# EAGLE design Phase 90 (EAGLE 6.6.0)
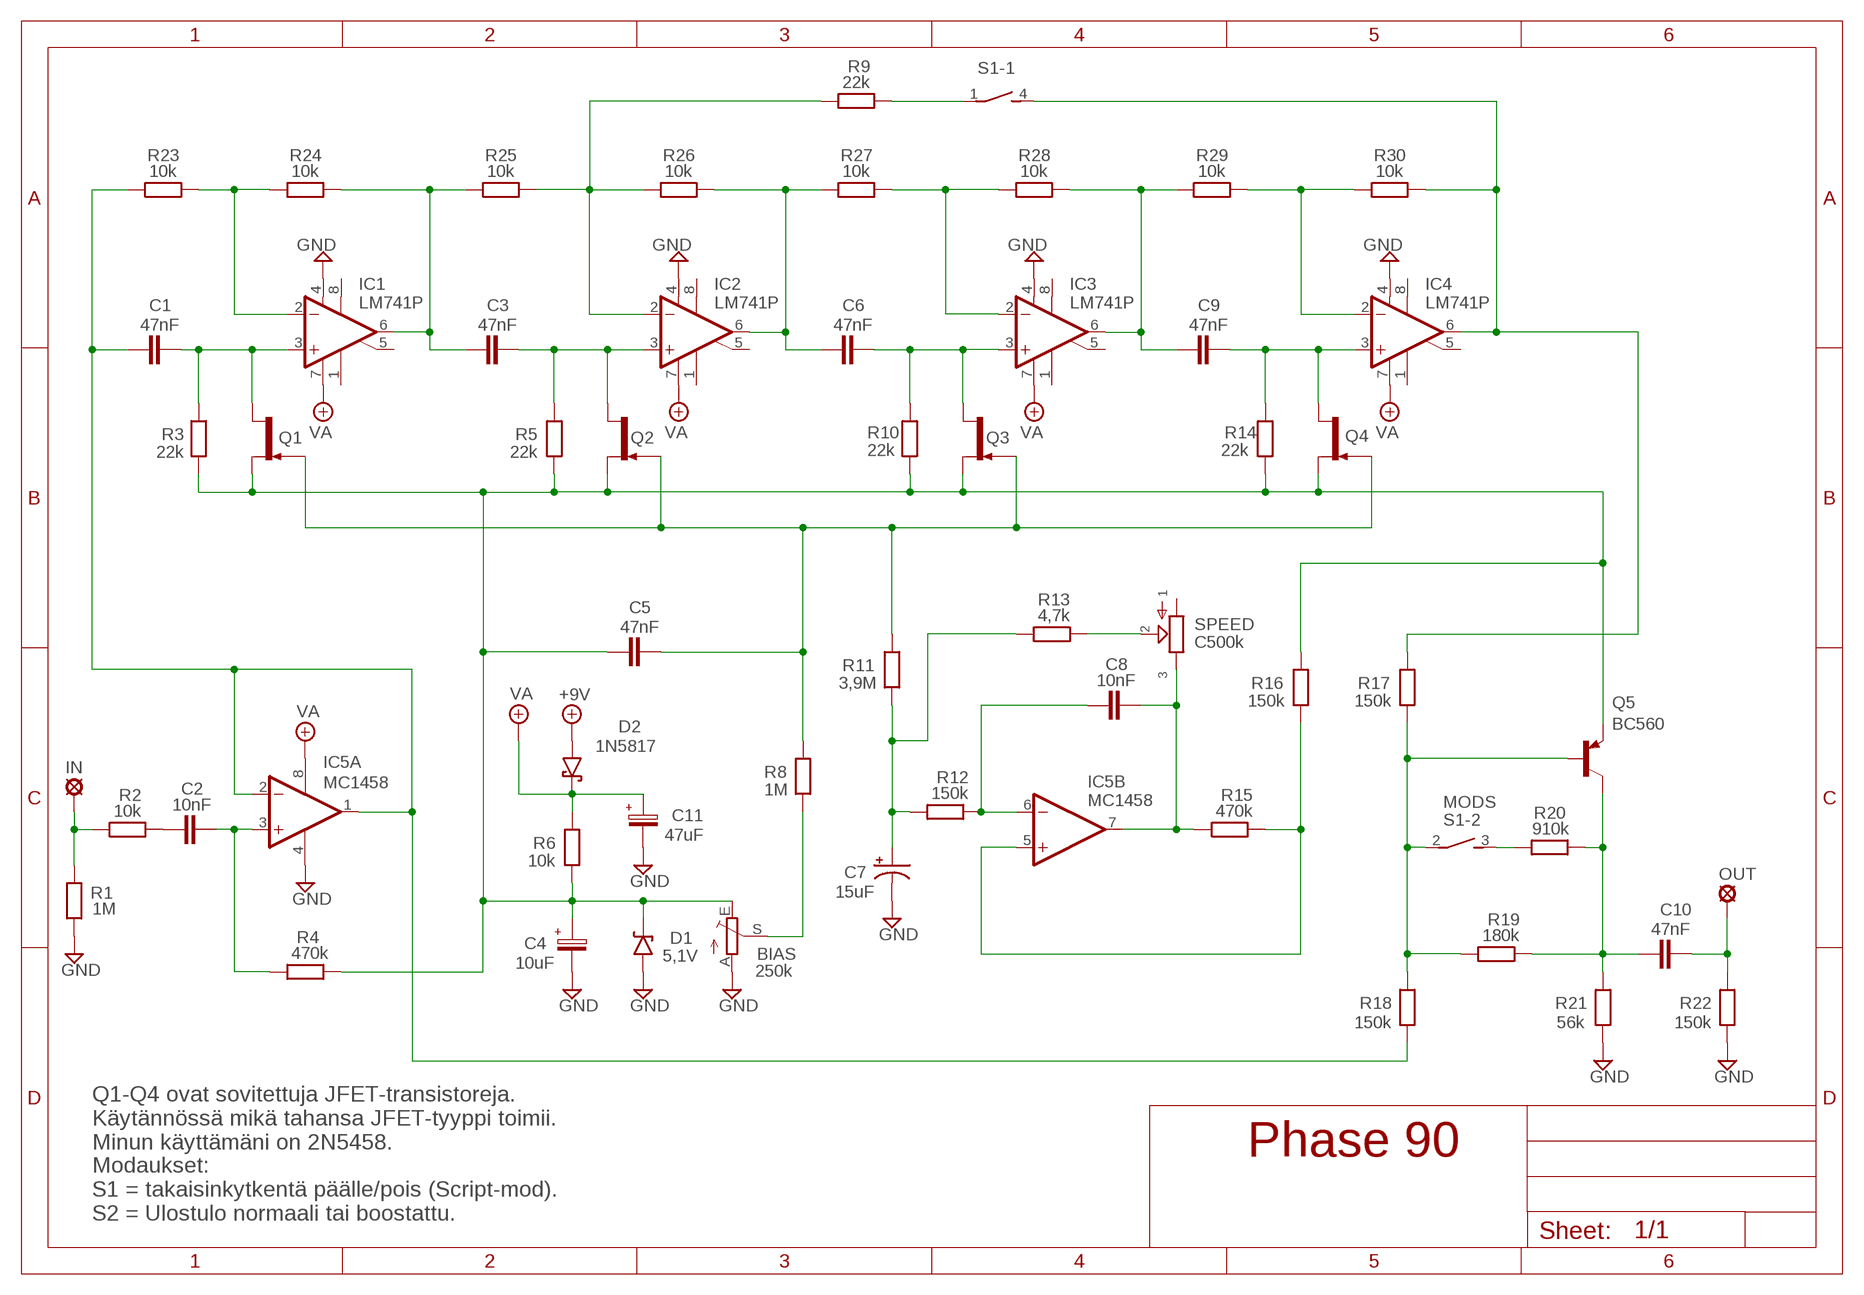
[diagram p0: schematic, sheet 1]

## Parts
+9V  +9V  +9V(T)1  [ROUND]
BIAS  250k  TRIM_EU-PT10  [PT-10]
C1  47nF  22NF-82NF"  [4,5MM]
C2  10nF  1NF-15NF  [3,5MM]
C3  47nF  22NF-82NF"  [4,5MM]
C4  10uF  063-EU  [063_025]
C5  47nF  22NF-82NF"  [4,5MM]
C6  47nF  22NF-82NF"  [4,5MM]
C7  15uF  044A2  [044A_2]
C8  10nF  1NF-15NF  [3,5MM]
C9  47nF  22NF-82NF"  [4,5MM]
C10  47nF  22NF-82NF"  [4,5MM]
C11  47uF  063-EU  [063_025]
D1  5,1V  1N9ZENER  [DO35-3]
D2  1N5817  [DO41-3]
GND  GND  GND(T)1  [ROUND]
GND5  GND  GND(T)1  [ROUND]
IC1  LM741P  [DIL08]
IC2  LM741P  [DIL08]
IC3  LM741P  [DIL08]
IC4  LM741P  [DIL08]
IC5  MC1458  TL072P  [DIL08]
IN  MCS10B  [MCS10B]
OUT  MCS10B  [MCS10B]
Q1  2N5457  [TO92-]
Q2  2N5457  [TO92-]
Q3  2N5457  [TO92-]
Q4  2N5457  [TO92-]
Q5  BC560  [TO92-EBC]
R1  1M  6MM-EU3  [R0207/3]
R2  10k  6MM-EU3  [R0207/3]
R3  22k  6MM-EU3  [R0207/3]
R4  470k  6MM-EU3  [R0207/3]
R5  22k  6MM-EU3  [R0207/3]
R6  10k  6MM-EU3  [R0207/3]
R8  1M  6MM-EU3  [R0207/3]
R9  22k  6MM-EU3  [R0207/3]
R10  22k  6MM-EU3  [R0207/3]
R11  3,9M  6MM-EU3  [R0207/3]
R12  150k  6MM-EU3  [R0207/3]
R13  4,7k  6MM-EU3  [R0207/3]
R14  22k  6MM-EU3  [R0207/3]
R15  470k  6MM-EU3  [R0207/3]
R16  150k  6MM-EU3  [R0207/3]
R17  150k  6MM-EU3  [R0207/3]
R18  150k  6MM-EU3  [R0207/3]
R19  180k  6MM-EU3  [R0207/3]
R20  910k  6MM-EU3  [R0207/3]
R21  56k  6MM-EU3  [R0207/3]
R22  150k  6MM-EU3  [R0207/3]
R23  10k  6MM-EU3  [R0207/3]
R24  10k  6MM-EU3  [R0207/3]
R25  10k  6MM-EU3  [R0207/3]
R26  10k  6MM-EU3  [R0207/3]
R27  10k  6MM-EU3  [R0207/3]
R28  10k  6MM-EU3  [R0207/3]
R29  10k  6MM-EU3  [R0207/3]
R30  10k  6MM-EU3  [R0207/3]
S1  MODS  DS02E  [DS-02]
SPEED  C500k  POT-EU16MM  [16MM]

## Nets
+9V: +9V.1(+9V) D2.A
GND: BIAS.A C4.- C7.2(-) C11.- D1.A GND5.1(GND) GND.1(GND) IC1.4(V-) IC2.4(V-) IC3.4(V-) IC4.4(V-) IC5.4(P:V-) R1.1 R21.1 R22.1
N$1: IC1.2(-IN) R23.2 R24.1
N$2: C1.2 IC1.3(+IN) Q1.3(D) R3.2
N$3: IC2.2(-IN) R9.1 R25.2 R26.1
N$4: C5.2 Q1.1(G) Q2.1(G) Q3.1(G) Q4.1(G) R8.2 R11.2
N$5: R20.1 S1.3
N$6: IC3.2(-IN) R27.2 R28.1
N$7: C3.1 IC1.6(OUT) R24.2 R25.1
N$8: C3.2 IC2.3(+IN) Q2.3(D) R5.2
N$9: R9.2 S1.1
N$10: C6.1 IC2.6(OUT) R26.2 R27.1
N$11: IC4.2(-IN) R29.2 R30.1
N$12: BIAS.S R8.1
N$13: C6.2 IC3.3(+IN) Q3.3(D) R10.2
N$14: C10.1 Q5.C R19.2 R20.2 R21.2
N$15: C9.2 IC4.3(+IN) Q4.3(D) R14.2
N$16: C9.1 IC3.6(OUT) R28.2 R29.1
N$17: IN.MP R1.2 R2.1
N$18: IC4.6(OUT) R17.2 R30.2 S1.4
N$19: C2.1 R2.2
N$20: C2.2 IC5.3(A:+IN) R4.1
N$21: C1.1 IC5.1(A:OUT) IC5.2(A:-IN) R18.1 R23.1
N$22: C10.2 OUT.MP R22.2
N$23: C8.2 IC5.7(B:OUT) R15.1 SPEED.3
N$24: IC5.5(B:+IN) R15.2 R16.1
N$25: C8.1 IC5.6(B:-IN) R12.2
N$26: C7.1(+) R11.1 R12.1 R13.1
N$27: R13.2 SPEED.2
N$28: Q5.B R17.1 R18.2 R19.1 S1.2
N$29: BIAS.E C4.+ C5.1 D1.C Q1.2(S) Q2.2(S) Q3.2(S) Q4.2(S) Q5.E R3.1 R4.2 R5.1 R6.1 R10.1 R14.1 R16.2
VA: C11.+ D2.C IC1.7(V+) IC2.7(V+) IC3.7(V+) IC4.7(V+) IC5.8(P:V+) R6.2
Unconnected: IC1.1(ON1) IC1.5(ON2) IC1.8(OPT) IC2.1(ON1) IC2.5(ON2) IC2.8(OPT) IC3.1(ON1) IC3.5(ON2) IC3.8(OPT) IC4.1(ON1) IC4.5(ON2) IC4.8(OPT) SPEED.1

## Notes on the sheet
- Q1-Q4 ovat sovitettuja JFET-transistoreja. 
  Käytännössä mikä tahansa JFET-tyyppi toimii.
  Minun käyttämäni on 2N5458.
- Modaukset:
  S1 = takaisinkytkentä päälle/pois (Script-mod).
  S2 = Ulostulo normaali tai boostattu.

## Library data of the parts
+9V = gm-supply:+9V(T): +9V Voltage Supply
BIAS = pot:TRIM_EU-: POTENTIOMETER
C1 C3 C5 C6 C9 C10 = Mylar Kondensaattorit:22NF-82NF: 22nF-82nF
C2 C8 = Mylar Kondensaattorit:1NF-15NF: 1nF-15nF
C4 C11 = Elektrolyytit:063-EU
C7 = Tantaalit:044A: .1 - 1.5µF
D1 = Diodit:1N9*ZENER: 1N9???B Zener Diode
D2 = Diodit:1N5817
GND GND5 = gm-supply:GND(T): Ground
IC1-IC4 = Operaatiovahvistimet:*741: OP AMP
IC5 = Operaatiovahvistimet:TL072: OP AMP
IN OUT = Padit:MCS10B: SOLDER PAD
Q1-Q4 = Transistorit:2N5457: N-CHANNEL JFET
Q5 = transistor-pnp:BC560*: PNP Transistror
R1-R6 R8-R30 = Vastukset:6MM-EU: 6mm Resistors (European schematic symbol)
S1 = switch-dil:DS02E: DIL/CODE SWITCH; OC_FARNELL: 9472126; OC_NEWARK: unknown
SPEED = gm-pots:POT-EU

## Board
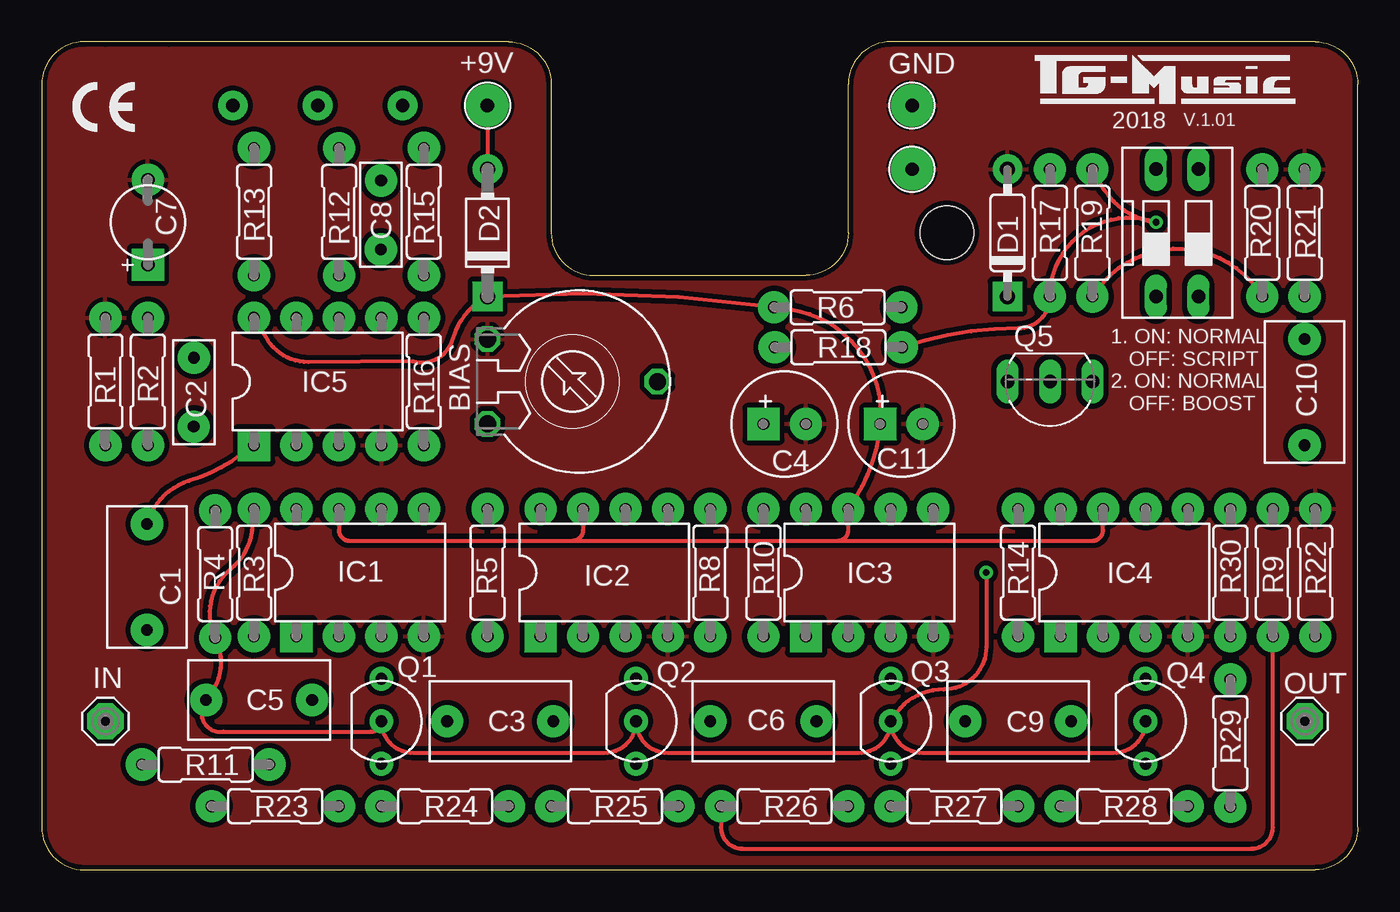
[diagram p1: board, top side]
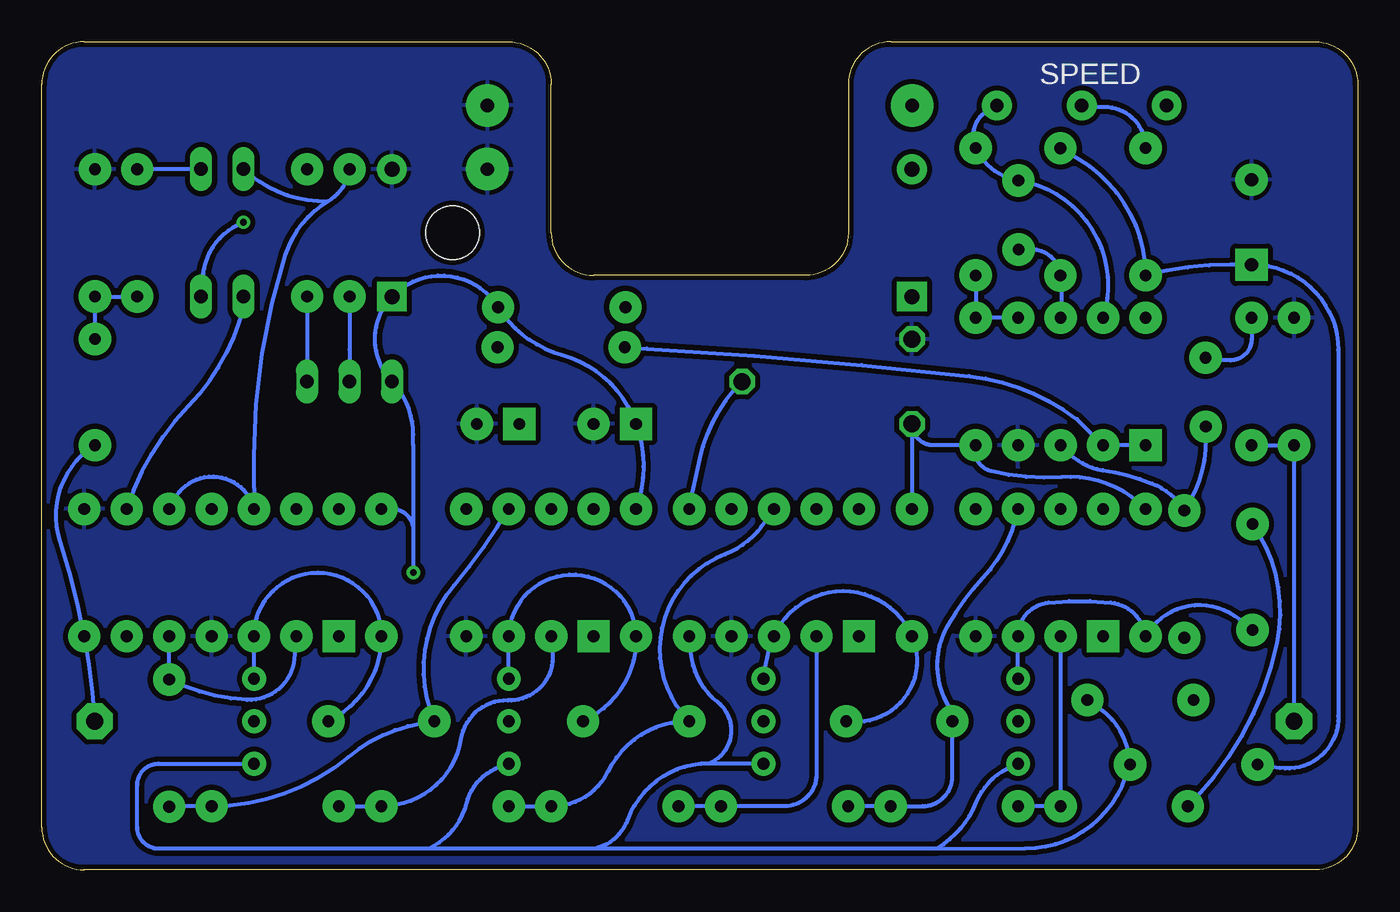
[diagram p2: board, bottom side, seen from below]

Size 78.74 x 49.53 mm. Coordinates in mm from the lower left corner, seen from the top.
Outline: 7.62,49.53 3.81,49.53
Outline: 78.74,2.54 78.74,46.99 arc90 76.2,49.53 50.8,49.53 arc90 48.26,46.99 48.26,38.1 arc-90 45.72,35.56 33.02,35.56 arc-90 30.48,38.1 30.48,46.99 arc90 27.94,49.53 2.54,49.53 arc90 0,46.99 0,2.54 arc90 2.54,0 76.2,0 arc90 78.74,2.54
Copper layers (1*16): Top 0.035mm / dielectric 1.5mm / Bottom 0.035mm
Design rules "ITEADstudio": minimum track width 10mil, minimum drill 12mil, track to track 12mil, track to pad 12mil, pad to pad 12mil, via to via 12mil, smd to smd 0mil, copper to edge 12mil, drill to drill 12mil, minimum pad ring 10mil, minimum via ring 6mil, stop-mask expansion 4mil, vias tented up to drill 100mil, thermal gap 10mil
Holes 3.2 mm at 54.16,38.11

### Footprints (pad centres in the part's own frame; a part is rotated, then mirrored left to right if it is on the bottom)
ROUND = drill 0.8 pad 2.54: 1 0,0
PT-10 = drill 1.016 octagon: A -2.54,-5.08; E 2.54,-5.08; S 0,5.08
4,5MM = drill 0.7 pad 1.93: 1 -3.175,0; 2 3.175,0
3,5MM = drill 0.7 pad 1.93: 1 -1.905,0; 2 2.221,-0.016
063_025 = drill 0.7 pad 1.93 square: + -1.27,0 | drill 0.7 pad 1.93: - 1.27,0
044A_2 = drill 0.8 pad 1.93 square: 1 -2.54,0 | drill 0.8 pad 1.93: 2 2.54,0
DO35-3 = drill 0.9 pad 1.778: A 3.81,0 | drill 0.9 pad 1.778 square: C -3.81,0
DO41-3 = drill 0.9 pad 1.778: A 3.81,0 | drill 0.9 pad 1.778 square: C -3.81,0
DIL08 = drill 0.7 pad 1.93 square: 1 -3.81,-3.81 | drill 0.7 pad 1.93: 2 -1.27,-3.81; 3 1.27,-3.81; 4 3.81,-3.81; 5 3.81,3.81; 6 1.27,3.81; 7 -1.27,3.81; 8 -3.81,3.81
MCS10B = drill 1.016 pad 2.159 octagon: MP 0,0
TO92- = drill 0.7 pad 1.422: 1 2.54,0; 2 0,0; 3 -2.54,0
TO92-EBC = drill 0.813 long: B 0,-1.27; C -2.54,-1.27; E 2.54,-1.27
R0207/3 = drill 0.7 pad 1.93: 1 -3.81,0; 2 3.81,0
DS-02 = drill 0.813 long: 1 -1.27,-3.81; 2 1.27,-3.81; 3 1.27,3.81; 4 -1.27,3.81
16MM = drill 0.8 pad 1.778: 1 5.08,0; 2 0,0; 3 -5.08,0

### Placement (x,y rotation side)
+9V  26.67,45.72 0 top
BIAS  31.75,29.21 270 top
C1  6.3,17.51 270 top
C2  9.11,28.73 270 top
C3  27.43,8.89 0 top
C4  44.45,26.67 0 top
C5  13.01,10.16 0 top
C6  43.18,8.89 0 top
C7  6.35,38.73 90 top
C8  20.29,39.02 90 top
C9  58.42,8.89 0 top
C10  75.56,28.57 270 top
C11  51.44,26.67 0 top
D1  57.78,38.1 90 top
D2  26.67,38.1 90 top
GND  52.07,45.72 0 top
GND5  52.07,41.91 0 top
IC1  19.05,17.78 0 top
IC2  33.66,17.78 0 top
IC3  49.53,17.78 0 top
IC4  64.77,17.78 0 top
IC5  16.51,29.21 0 top
IN  3.81,8.89 0 top
OUT  75.56,8.89 0 top
Q1  20.32,8.89 270 top
Q2  35.56,8.89 270 top
Q3  50.8,8.89 270 top
Q4  66.04,8.89 270 top
Q5  60.33,27.94 180 top
R1  3.81,29.21 270 top
R2  6.35,29.21 90 top
R3  12.7,17.78 270 top
R4  10.38,17.69 270 top
R5  26.67,17.78 270 top
R6  47.62,33.66 180 top
R8  40.01,17.78 270 top
R9  73.66,17.78 90 top
R10  43.18,17.78 270 top
R11  9.81,6.3 0 top
R12  17.79,39.35 270 top
R13  12.7,39.37 90 top
R14  58.42,17.78 270 top
R15  22.86,39.37 270 top
R16  22.86,29.21 270 top
R17  60.33,38.1 90 top
R18  47.66,31.26 0 top
R19  62.87,38.1 270 top
R20  73.03,38.1 270 top
R21  75.56,38.1 270 top
R22  76.2,17.78 270 top
R23  13.97,3.81 0 top
R24  24.13,3.81 0 top
R25  34.29,3.81 0 top
R26  44.45,3.81 0 top
R27  54.61,3.81 0 top
R28  64.77,3.81 0 top
R29  71.12,7.58 90 top
R30  71.12,17.78 90 top
S1  67.94,38.1 0 top
SPEED  16.51,45.72 0 bottom

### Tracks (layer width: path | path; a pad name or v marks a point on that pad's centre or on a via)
+9V
  Top 0.254: +9V.1 D2.A
GND
  pour Bottom: 0,2.46 0,46.99 arc-90 2.54,49.53 27.94,49.53 arc-90 30.48,46.99 30.48,37.93 arc90 32.85,35.56 45.72,35.56 arc90 48.26,38.1 48.26,46.99 arc-90 50.8,49.53 76.2,49.53 arc-90 78.74,46.99 78.74,2.45 arc-90 76.29,0 2.46,0 arc-90
  pour Top: 0,2.48 0,46.99 arc-90 2.54,49.53 27.94,49.53 arc-90 30.48,46.99 30.48,38.01 arc90 32.93,35.56 45.72,35.56 arc90 48.26,38.1 48.26,46.99 arc-90 50.8,49.53 76.2,49.53 arc-90 78.74,46.99 78.74,2.46 arc-90 76.28,0 2.48,0 arc-90
N$1
  Bottom 0.254: R24.1 R23.2 IC1.2
N$2
  Bottom 0.254: Q1.3 IC1.3 arc84 18.5,15.99 arc12 14.78,15.99 arc76 R3.2 arc99 7.08,14.98 C1.2
N$3
  Top 0.254: R26.1 40.64,2.54 arc90 41.91,1.27 72.39,1.27 arc90 73.66,2.54 R9.1
  Bottom 0.254: IC2.2 32.38,5.71 arc90 34.29,3.81 R25.2 R26.1
N$4
  Bottom 0.254: 25.4,1.27 25.17,1.27 arc-36 22.83,4.04 arc42 20.99,6.02 Q1.1 | 25.4,1.27 45.62,1.27 | 45.62,1.27 55.56,1.27 | Q2.1 37.47,6.35 38.82,6.36 | 55.56,1.27 71.75,1.27 arc90 73.03,2.54 73.03,5.08 arc90 71.75,6.35 Q4.1 | 38.82,6.36 arc-70 43.69,2.99 arc56 45.62,1.27 | Q3.1 51.36,6.15 arc-55 53.35,3.96 arc49 55.56,1.27 | 25.4,1.27 19.89,1.28 arc-65 14.09,5.02 R11.2 arc-53 15.63,9.79 C5.2 | R8.2 39.91,12.97 arc-47 38.32,10.06 arc119 38.82,6.36
N$5
  Bottom 0.254: S1.3 R20.1
N$6
  Bottom 0.254: R28.1 R27.2 arc-81 53.67,7.81 arc82 50.86,10.13 arc-29 49.55,10.44 arc-67 48.17,12.94 IC3.2
N$7
  Bottom 0.254: R25.1 R24.2 26.04,3.81 arc-90 24.26,5.59 C3.1 arc-30 24.52,9.87 arc60 24.52,14.63 arc13 22.41,17.47 arc-32 IC1.6
N$8
  Bottom 0.254: Q2.3 35.42,12.3 arc14 IC2.3 arc133 R5.2 arc122 C3.2
N$9
  Bottom 0.254: S1.1 66.67,33.66 arc30 69.97,27.73 arc-26 R9.2
N$10
  Bottom 0.254: R27.1 48.47,3.81 | 48.47,3.81 R26.2 | 48.47,3.81 arc-68 44.89,5.85 arc64 C6.1 arc114 37.85,18.88 arc-33 35.68,20.55 IC2.6
N$11
  Bottom 0.254: R30.1 arc90 R30.1 R29.2 arc-24 66.45,10.17 arc-87 63.63,12.62 IC4.2
N$12
  Bottom 0.254: R8.1 39.36,24.59 arc33 BIAS.S
N$13
  Bottom 0.254: Q3.3 50.81,12.13 arc3 IC3.3 arc176 R10.2 arc68 C6.2
N$14
  Top 0.254: R19.2 63.23,34.79 arc-112 R20.2
  Bottom 0.254: R19.2 Q5.C | R20.2 R21.2 C10.1
N$15
  Bottom 0.254: Q4.3 IC4.3 arc180 R14.2 arc64 C9.2
N$16
  Bottom 0.254: R29.1 arc90 71.08,3.81 R28.2 arc-40 60.39,6.76 arc34 C9.1 arc64 54.08,17.02 arc-7 51.49,20.52 IC3.6
N$17
  Bottom 0.254: IN.MP R1.2 R2.1
N$18
  Bottom 0.254: 61.59,40.01 arc-41 64.14,36.83 arc-18 66.04,24.77 66.04,22.86 IC4.6 arc-137 70.81,22.17 R30.2 | 61.59,40.01 arc-51 R17.2 | S1.4 66.23,41.55 arc-41 61.59,40.01
N$19
  Bottom 0.254: R2.2 6.35,31.75 arc90 7.62,30.48 8.95,30.48 arc90 C2.1
N$20
  Bottom 0.254: C2.2 9.09,25.82 arc34 R4.1 arc-37 12.29,23.11 arc-13 15.27,23.91 arc35 17.24,24.89 IC5.3
N$21
  Top 0.254: IC5.1 11.91,24.82 arc-20 8.81,23.27 arc58 C1.1
  Bottom 0.254: IC5.1 IC5.2 16.8,26.96 arc-31 23.25,29.53 arc-3 42.54,31.18 R18.1 | R23.1 9.6,4.4 arc-32 4.82,13.59 arc-47 C1.1
N$22
  Bottom 0.254: C10.2 arc-76 77.64,19.64 arc8 R22.2 arc6 OUT.MP
N$23
  Bottom 0.254: SPEED.3 22.11,45.44 arc-86 R15.1 arc-56 C8.2 arc99 IC5.7
N$24
  Bottom 0.254: R15.2 R16.1 IC5.5
N$25
  Bottom 0.254: C8.1 19.54,37.12 arc85 R12.2 arc10 IC5.6
N$26
  Bottom 0.254: R12.1 16.67,42.49 arc58 R13.1 arc14 7.62,36.2 C7.1 6.27,36.2 arc90 1.16,31.09 1.16,9.21 arc100 4.66,6.1 R11.1
N$27
  Bottom 0.254: SPEED.2 15.78,45.72 arc90 15.71,45.64 15.16,45.64 arc90 R13.2
N$28  (via drill 0.4 pad 0.8)
  Top 0.254: R18.2 arc-18 58.42,32.38 arc90 R17.1 arc-110 v66.67,38.73 arc-54 63.37,40.99 R19.1
  Bottom 0.254: R17.1 60.33,31.11 Q5.B | S1.2 69.07,35.62 arc63 v66.67,38.73
N$29  (via drill 0.4 pad 0.8)
  Top 0.254: Q3.2 arc-90 48.9,6.99 37.47,6.99 arc-90 Q2.2 arc-90 33.66,6.99 22.23,6.99 arc-90 Q1.2 arc-90 19.68,8.26 19.68,8.27 10.88,8.27 arc-142 9.85,10.14 C5.1 arc68 R4.2 arc-77 11.29,17.98 arc45 12.57,20.35 R3.1 | Q4.2 arc-90 64.14,6.99 52.7,6.99 arc-90 Q3.2 | v56.52,17.78 56.52,13.34 arc-90 53.98,10.79 arc62 Q3.2
  Bottom 0.254: R5.1 BIAS.E arc-90 25.4,25.4 R16.2 arc-91 21.93,23.84 arc-18 17.72,23.5 arc50 12.73,21.62 R3.1 | 56.52,20.32 56.52,25.4 56.52,26.04 arc-44 Q5.E arc87 D1.C arc104 R6.1 arc-42 47.61,30.8 arc55 C4.+ arc39 R10.1 | R14.1 57.78,21.59 arc90 56.52,20.32 | 56.52,20.32 v56.52,17.78
VA
  Top 0.254: IC1.7 17.78,20.32 arc90 18.41,19.68 23.5,19.68 31.11,19.68 31.75,19.68 | 31.75,19.68 32.38,19.68 47.62,19.68 | 47.62,19.68 arc90 48.26,20.32 IC3.7 arc30 C11.+ arc88 44.77,33.52 R6.2 arc12 D2.C arc41 24.76,32.24 24.49,31.54 arc-85 22.2,30.41 15.95,30.37 arc-62 13.39,31.89 IC5.8 | 47.62,19.68 62.87,19.68 arc90 63.5,20.32 IC4.7 | IC2.7 32.38,20.32 arc-90 31.75,19.68

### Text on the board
tNames: 2018 | V.1.01 | 1. ON: NORMAL / OFF: SCRIPT / 2. ON: NORMAL / OFF: BOOST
